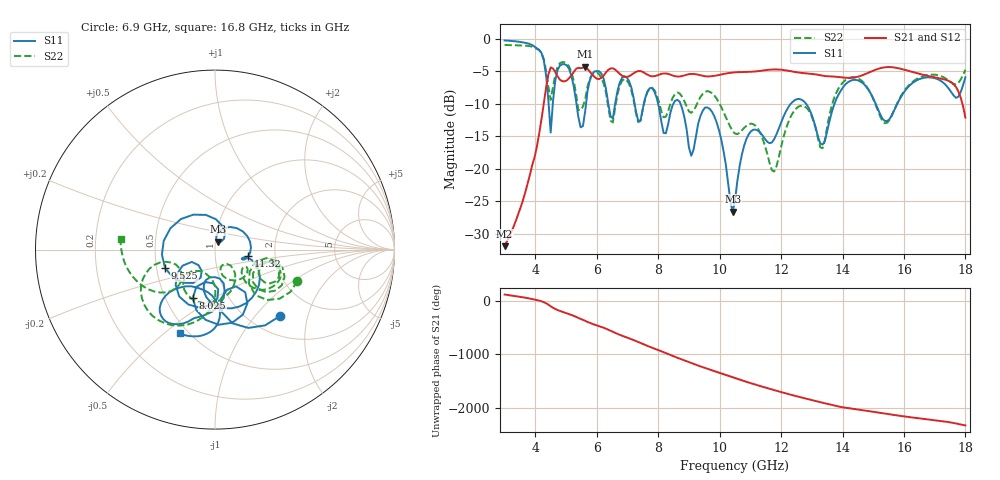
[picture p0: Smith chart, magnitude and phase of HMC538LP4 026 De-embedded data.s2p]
! Chelmsford, MA 01824
! http://www.hittite.com
! Tel: 978-250-3343
! Fax: 978-250-3373
! Device  :  HMC538LP4
! Description:  600 Analog Phase Shifter
! Frequency  :  6.0 GHz - 15.0 GHz
! Package  :  LP4  - 4x4 mm Quad Flatpack No-Lead (QFN) Plastic Package: 24 pin
! Ports  :  2 RF, 1 DC
!  Pin  3  = Rfin  = Port 1
!  Pin  16  = Rfout = Port 2
!  pin  21  = vCTL
! Voltages:  VCTL  = 0 to 5.0 Volts
! Currents :  Vb(V)  Vd(V)  Ib(mA)  Id(mA)
!  0.00  2.60  0.000000	0.471880
! Data:  The device was measured on evaluation board 111296-1.
!  Data was collected using a calibrated network analyzer.
!  The evaluation circuit board was modeled and simulated.This was use
!  to removed the evaluation board circuit from the measured data.
!  The reference plane is the center of the package pin.
! Misc:  Lot #
!Date Measured:  03 - 11 -2009
! Date:  03 - 17 -2009
! Note:
!  Hittite Microwave supplies this data as a sample of measured data at the
!  package pin for this package product.  Your particular data for this product
!  may vary.
!  Data was taken at 25 degrees C.
!  Hittite Microwave reserves the right to change this data at anytime.
# MHz S MA R 50
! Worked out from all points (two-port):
!   201 points, 3 GHz to 18 GHz, reference 50 ohm
!   highest |S21| = -4.26 dB at 5.625 GHz (marker M1); lowest = -31.9 dB at 3 GHz (marker M2)
!   |S21| within 3 dB of the highest: 4.359 GHz to 17.67 GHz (13.31 GHz wide, 121 % of centre)
!   lowest |S11| = -26.6 dB at 10.43 GHz (marker M3), VSWR 1.10, Z = 51.6 + j4.49 ohm
!   |S11| at or under -10 dB: 8.726 GHz to 12.31 GHz (3.585 GHz wide, 34.1 % of centre); 12.82 GHz to 13.74 GHz (918.4 MHz wide, 6.92 % of centre); 15.08 GHz to 15.78 GHz (700 MHz wide, 4.54 % of centre)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
!   |S22| runs from -20.4 to -0.9 dB; largest |S21 - S12| = 0.0013
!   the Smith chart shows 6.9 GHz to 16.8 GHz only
!   S11 on the Smith chart (normalised r, x): 6.9 GHz: 1.35, -1.36; 8.025 GHz: 0.68, -0.40; 9.525 GHz: 0.55, -0.13; 11.32 GHz: 1.45, -0.11; 16.8 GHz: 0.45, -0.57
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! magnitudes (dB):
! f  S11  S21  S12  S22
! 3 GHz  -0.2  -31.9  -31.9  -0.9
! 4.2 GHz  -2.2  -12.4  -12.4  -2.1
! 4.5 GHz  -14.4  -4.4  -4.4  -9.4
! 4.875 GHz  -3.9  -6.5  -6.5  -3.6
! 5.55 GHz  -13.4  -4.4  -4.4  -10.4
! 5.625 GHz  -11.0  -4.3  -4.3  -9.2
! 6.075 GHz  -5.0  -6.2  -6.2  -5.4
! 6.525 GHz  -12.2  -4.5  -4.5  -12.8
! 6.9 GHz  -5.7  -5.8  -5.8  -6.2
! 8.025 GHz  -10.5  -5.5  -5.5  -9.7
! 9.075 GHz  -18.0  -5.4  -5.4  -11.4
! 9.525 GHz  -10.6  -5.7  -5.7  -8.2
! 10.43 GHz  -26.6  -5.2  -5.2  -14.2
! 10.5 GHz  -24.9  -5.1  -5.1  -14.6
! 11.32 GHz  -14.4  -4.9  -4.9  -14.5
! 11.78 GHz  -15.4  -4.7  -4.7  -20.4
! 13.05 GHz  -12.4  -5.4  -5.4  -12.6
! 13.35 GHz  -16.3  -5.7  -5.7  -16.8
! 14.32 GHz  -6.3  -6.0  -6.0  -5.9
! 15.53 GHz  -12.4  -4.3  -4.3  -12.5
! 16.8 GHz  -5.9  -5.7  -5.7  -5.5
! 18 GHz  -5.9  -12.1  -12.1  -4.7
